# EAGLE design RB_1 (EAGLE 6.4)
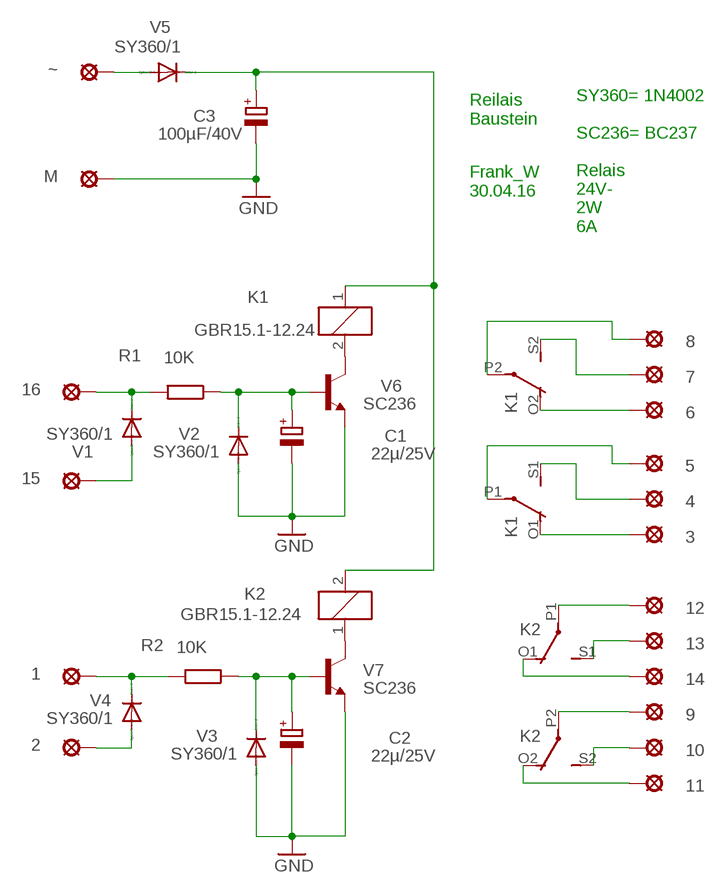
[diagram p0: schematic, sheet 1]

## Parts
1  LSP10  [LSP10]
2  LSP10  [LSP10]
3  LSP10  [LSP10]
4  LSP10  [LSP10]
5  LSP10  [LSP10]
6  LSP10  [LSP10]
7  LSP10  [LSP10]
8  LSP10  [LSP10]
9  LSP10  [LSP10]
10  LSP10  [LSP10]
11  LSP10  [LSP10]
12  LSP10  [LSP10]
13  LSP10  [LSP10]
14  LSP10  [LSP10]
15  LSP10  [LSP10]
16  LSP10  [LSP10]
C1  22µ/25V  CPOL-EUE5-5  [E5-5]
C2  22µ/25V  CPOL-EUE5-5  [E5-5]
C3  100µF/40V  CPOL-EUE22-9AXIAL  [E22-9]
K1  GBR15.1-12.24  4052  [F4052]
K2  GBR15.1-12.24  4052  [F4052]
M  LSP10  [LSP10]
R1  10K  R-EU_0207/12  [0207/12]
R2  10K  R-EU_0207/12  [0207/12]
V1  SY360/1  1N4004  [DO41-10]
V2  SY360/1  1N4004  [DO41-10]
V3  SY360/1  1N4004  [DO41-10]
V4  SY360/1  1N4004  [DO41-10]
V5  SY360/1  1N4004  [DO41-10]
V6  SC236  BC237  [TO92]
V7  SC236  BC237  [TO92]
~  LSP10  [LSP10]

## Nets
GND: C1.- C2.- C3.- M.MP V2.A V3.A V6.1(E) V7.1(E)
N$1: V5.A ~.MP
N$2: 13.MP K2.S1(2:S)
N$3: 12.MP K2.P1(2:P)
N$4: 14.MP K2.O1(2:O)
N$5: 9.MP K2.P2(3:P)
N$6: 10.MP K2.S2(3:S)
N$7: 11.MP K2.O2(3:O)
N$8: K2.1 V7.3(C)
N$9: 3.MP K1.O1(2:O)
N$10: C3.+ K1.1 K2.2 V5.C
N$11: 16.MP R1.2 V1.C
N$12: K1.2 V6.3(C)
N$13: 1.MP R2.2 V4.C
N$14: 2.MP V4.A
N$15: 4.MP K1.S1(2:S)
N$16: 5.MP K1.P1(2:P)
N$17: 6.MP K1.O2(3:O)
N$18: 7.MP K1.S2(3:S)
N$19: 8.MP K1.P2(3:P)
N$20: C2.+ R2.1 V3.C V7.2(B)
N$21: 15.MP V1.A
N$23: C1.+ R1.1 V2.C V6.2(B)

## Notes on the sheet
- Reilais
  Baustein
- Frank_W
  30.04.16
- SY360= 1N4002
  
  SC236= BC237
  
  Relais
  24V-
  2W
  6A

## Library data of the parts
1-16 M ~ = solpad:LSP10: SOLDER PAD
C1-C3 = rcl:CPOL-EU: POLARIZED CAPACITOR, European symbol
K1 K2 = relay:4052: RELAY 2 x switch, Finder; OC_FARNELL: unknown; OC_NEWARK: unknown
R1 R2 = rcl:R-EU_: RESISTOR, European symbol
V1-V5 = diode:1N4004: DIODE
V6 V7 = transistor-neu-to92:BC237: NPN TRANSISTOR

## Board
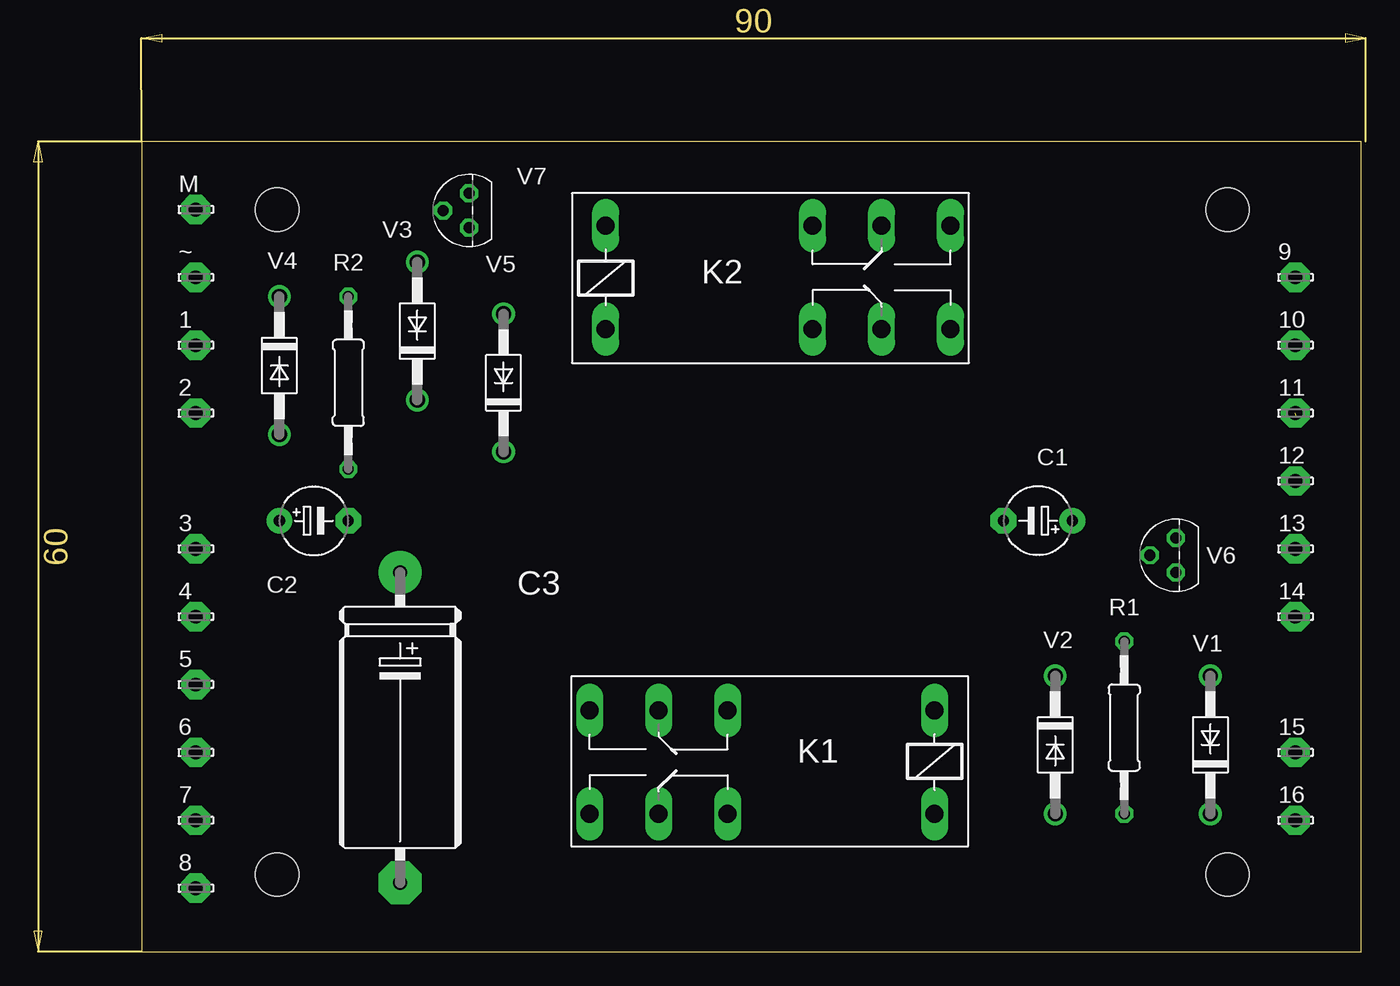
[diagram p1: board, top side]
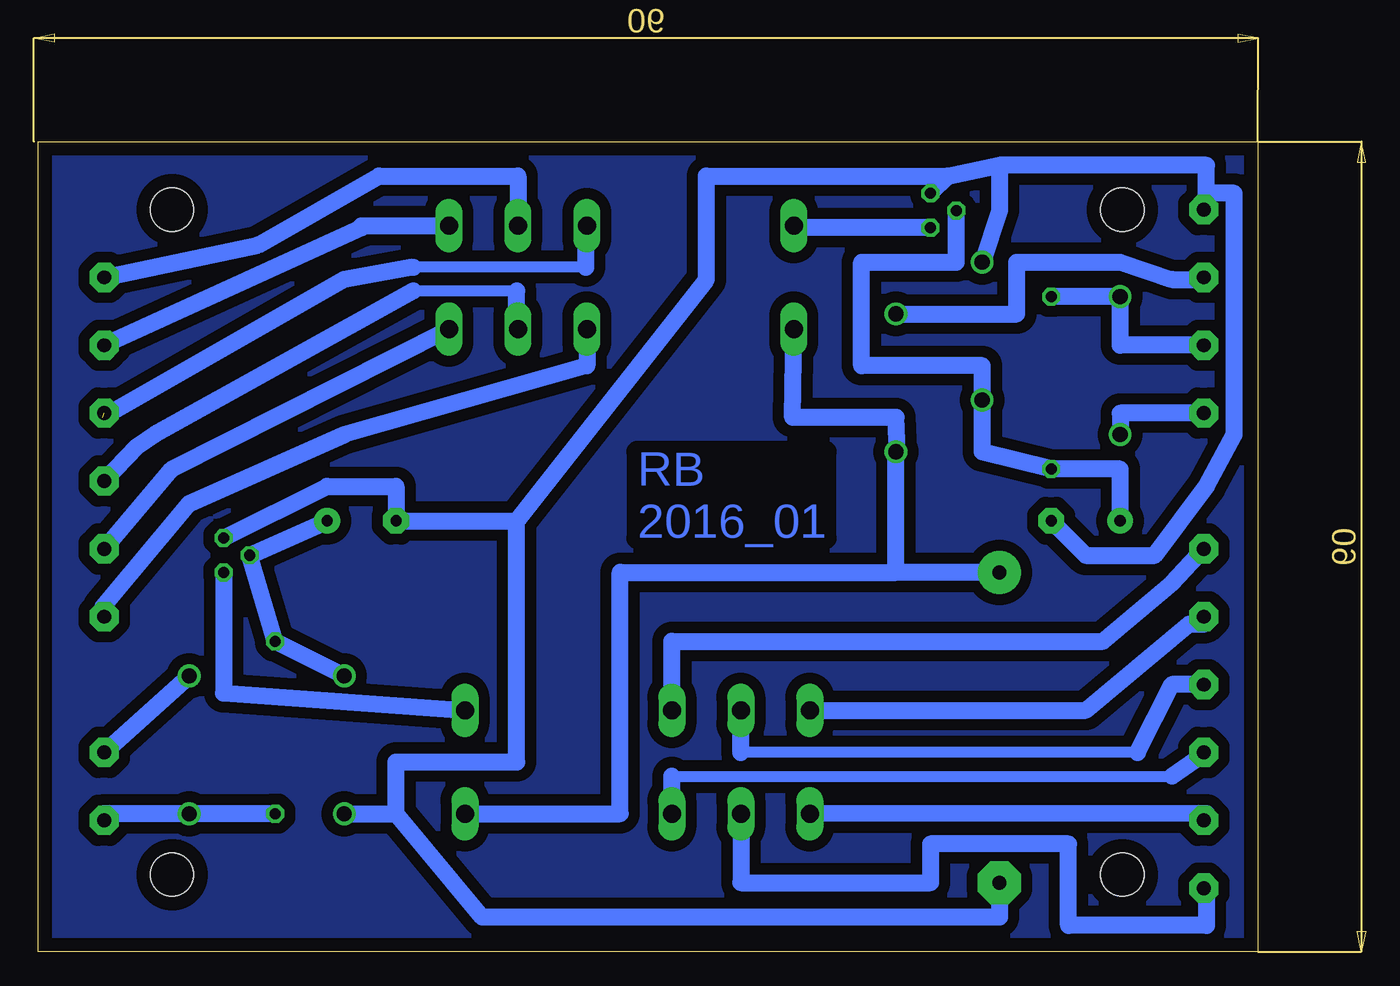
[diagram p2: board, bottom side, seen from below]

Size 98.09 x 67.61 mm. Coordinates in mm from the lower left corner, seen from the top.
Outline: 7.92,0 97.76,0 97.76,59.68 7.92,59.68 7.92,0
Copper layers (1*16): Top 0.035mm / dielectric 1.5mm / Bottom 0.035mm
Design rules "default *": minimum track width 20mil, minimum drill 24mil, track to track 8mil, track to pad 8mil, pad to pad 8mil, via to via 8mil, smd to smd 8mil, copper to edge 40mil, drill to drill 8mil, minimum pad ring 10mil, minimum via ring 8mil, stop-mask expansion 4mil, vias tented up to drill 0mil, thermal gap 20mil
Holes 3.2 mm at 87.92,54.68 87.92,5.68 17.92,5.68 17.92,54.68

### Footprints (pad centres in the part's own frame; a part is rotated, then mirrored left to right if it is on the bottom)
LSP10 = drill 1.016 pad 2.159 octagon: MP 0,0
E5-5 = drill 0.813 pad 1.905: + -2.54,0 | drill 0.813 pad 1.905 octagon: - 2.54,0
E22-9 = drill 1.016 pad 3.15: + -11.43,0 | drill 1.016 pad 3.15 octagon: - 11.43,0
F4052 = drill 1.321 long: 1 -3.81,3.81; 2 -3.81,-3.81; O1 11.43,-3.81; O2 11.43,3.81; P1 16.51,-3.81; P2 16.51,3.81; S1 21.59,-3.81; S2 21.59,3.81
0207/12 = drill 0.813 octagon: 1 -6.35,0; 2 6.35,0
DO41-10 = drill 1.118: A 5.08,0; C -5.08,0
TO92 = drill 0.813 octagon: 1 1.27,0; 2 0,1.905; 3 -1.27,0

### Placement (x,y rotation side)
1  11.92,44.68 0 top
2  11.92,39.68 0 top
3  11.92,29.68 0 top
4  11.92,24.68 0 top
5  11.92,19.68 0 top
6  11.92,14.68 0 top
7  11.92,9.68 0 top
8  11.92,4.68 0 top
9  92.92,49.68 0 top
10  92.92,44.68 0 top
11  92.92,39.68 0 top
12  92.92,34.68 0 top
13  92.92,29.68 0 top
14  92.92,24.68 0 top
15  92.92,14.68 0 top
16  92.92,9.68 0 top
C1  73.96,31.75 180 top
C2  20.62,31.75 0 top
C3  26.97,16.51 270 top
K1  62.53,13.97 180 top
K2  45.92,49.68 0 top
M  11.92,54.68 0 top
R1  80.31,16.51 270 top
R2  23.16,41.91 90 top
V1  86.66,15.24 90 top
V2  75.23,15.24 270 top
V3  28.24,45.72 90 top
V4  18.08,43.18 270 top
V5  34.59,41.91 90 top
V6  84.12,29.21 90 top
V7  32.05,54.61 90 top
~  11.92,49.68 0 top

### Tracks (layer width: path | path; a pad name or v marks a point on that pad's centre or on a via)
GND
  Bottom 1.27: M.MP 11.73,54.68 11.73,55.88 | 11.73,55.88 11.73,57.93 26.97,57.93 | 26.97,57.93 26.97,54.61 V3.A | V7.1 30.78,57.15 | 30.78,57.15 26.97,57.93 | C2.- 20.62,29.21 15.54,29.21 11.73,34.29 9.67,38.1 9.67,55.88 11.73,55.88 | C3.- 26.97,2.54 65.07,2.54 71.42,10.16 | 71.42,10.16 71.42,13.97 62.53,13.97 62.53,31.75 | 62.53,31.75 48.56,49.53 48.56,57.15 30.78,57.15 | 62.53,31.75 C1.- 71.42,34.29 76.5,34.29 V6.1 | V2.A 71.42,10.16
N$1
  Bottom 1.27: V5.A 25.7,46.99 25.7,50.8 18.08,50.8 14.27,49.53 11.92,49.53 ~.MP
N$2
  Bottom 1.27: 13.MP 87.93,35.56 K2.S1
N$3
  Bottom 0.813: 62.53,48.68 70.15,48.68
  Bottom 1.27: K2.P1 62.53,45.87 62.53,48.68 | 70.15,48.68 89.2,38.1 90.47,37.22 12.MP
N$4
  Bottom 1.27: K2.O1 57.35,43.18 75.23,38.1 86.66,33.02 93.01,25.4 92.92,25.4 14.MP
N$5
  Bottom 1.27: 9.MP 81.58,52.07 72.69,57.15 62.43,57.15 K2.P2
N$6
  Bottom 1.27: 10.MP 73.96,53.34 73.96,53.49 K2.S2
N$7  (1 unrouted)
  Bottom 0.813: 57.45,50.43 70.15,50.43
  Bottom 1.27: K2.O2 57.45,53.49 57.45,50.43 | 70.15,50.43 75.23,49.53 93.01,39.37
N$8
  Bottom 1.27: V7.3 42.11,53.34 K2.1
N$9
  Bottom 1.27: K1.O1 51.1,22.86 19.35,22.86 14.27,27.14 3.MP
N$10
  Bottom 1.27: C3.+ 34.59,27.94 | 34.59,27.94 V5.C 34.49,36.83 34.59,39.37 42.21,39.37 K2.2 | K1.1 54.91,10.16 54.91,27.94 34.59,27.94
N$11
  Bottom 1.27: R1.2 V1.C 92.92,10.16 16.MP
N$12
  Bottom 1.27: V6.3 84.12,19.05 K1.2
N$13
  Bottom 1.27: 1.MP 18.08,44.68 V4.C R2.2
N$14
  Bottom 1.27: 2.MP 18.08,39.68 V4.A
N$15
  Bottom 1.27: K1.S1 20.62,17.78 13,24.13 11.92,24.13 4.MP
N$16
  Bottom 0.813: 16.81,14.68 46.02,14.68
  Bottom 1.27: 5.MP 14.27,19.68 16.81,14.68 | 46.02,14.68 K1.P1
N$17
  Bottom 0.813: 51.1,12.93 14.27,12.93
  Bottom 1.27: K1.O2 51.1,12.93 | 6.MP 11.73,14.68 14.27,12.93
N$18
  Bottom 1.27: 7.MP 11.73,9.68 11.73,10.16 40.94,10.18 K1.S2
N$19
  Bottom 1.27: K1.P2 46.02,5.08 32.05,5.08 32.05,7.93 21.89,7.93 21.89,1.93 11.73,1.93 11.73,4.68 8.MP
N$20
  Bottom 1.27: C2.+ 18.08,35.56 R2.1 28.24,36.83 V3.C 28.24,43.18 37.13,43.18 37.13,50.8 30.15,50.8 V7.2
N$21
  Bottom 1.27: 15.MP V1.A
N$22
  pour Bottom (isolate 0.813): 7.92,59.69 98.09,59.69 98.09,0 7.92,0
N$23
  Bottom 1.27: V2.C R1.1 V6.2 C1.+

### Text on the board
Bottom: RB / 2016_01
